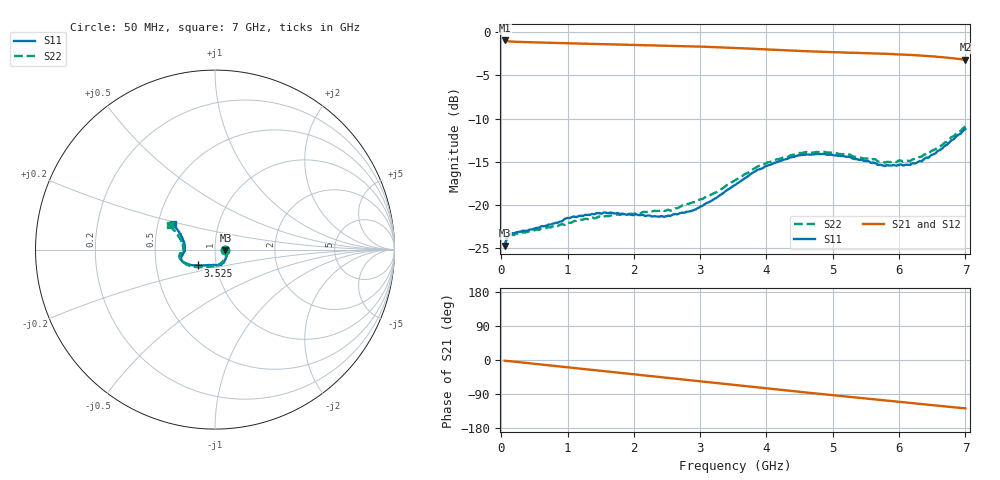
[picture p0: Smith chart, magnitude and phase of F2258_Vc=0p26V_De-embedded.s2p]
! Integrated Device Technology
! Corporate Headquarters
! 6024 Silver Creek Valley Road
! San Jose, CA 95138  USA
! Phone:  1-408-284-8200
! Toll Free:  1-800-223-1366
! Webpage:  http://www.idt.com/
! Timing and RF Division
! 515 Groton Road, Suite 102
! Westford, MA 01886-6024
! Device:  F2258
! Description: Voltage Variable RF Attenuator
! Frequency:  50.0 -  6000.00 MHz
! Package:  3x3 mm Thin QFN Plastic Package: 16 pin
! Ports:  2 RF, 2 DC
!  Pin  1  = NC
!  Pin  2  = NC
!  Pin  3  = RF2  = Port 2
!  Pin  4  = GND
!  Pin  5  = Vdd
!  Pin  6  = NC
!  Pin  7  = VCTRL
!  Pin  8  = NC
!  Pin  9  = GND
!  Pin 10  = RF1  = Port 1
!  Pin 11  = NC
!  Pin 12  = NC
!  Pin 13  = NC
!  Pin 14  = NC
!  Pin 15  = NC
!  Pin 16  = NC
! Vcntrl:  0.260 Volts
! Vdd:  +3.300 Volts
! Current:  1.080 mA
! Data:  The device was measured on a the F2258 evaluation board which has
!  individual transmission lines to the RF pins.  Data was collected
!  using a calibrated network analyzer.  The evaluation board was
!  de-embedded using a TRL calibration technique.
!  The reference plane is the edge of the package pin.
! Misc:  SN 10
!  Action Tracker AT0285
! Date Measured:  2014-12-10
! Date:  2016-01-13  MJV
! Note:
!  Integrated Device Technology supplies this data as a sample of measured
!  data at the package pin for this product.  Your particular data for this
!  product may vary.
!  Data was taken at 25 degrees C.
!  Integrated Device Technology reserves the right to change this data at anytime.
!Freq_(GHz)  S11M_(dB)  S11P_(deg)  S21M_(dB)  S21P_(deg)  S12M_(dB)  S12P_(deg)  S22M_(dB)  S22P_(deg)
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# GHz S dB R 50
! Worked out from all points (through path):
!   201 points, 50 MHz to 7 GHz, reference 50 ohm
!   highest |S21| = -0.97 dB at 50 MHz (marker M1); lowest = -3.2 dB at 7 GHz (marker M2)
!   group delay of S21, straight-line fit = 50.5 ps
!   lowest |S11| = -24.7 dB at 50 MHz (marker M3), VSWR 1.12, Z = 56.2 - j0.392 ohm
!   |S11| at or under -10 dB: start of sweep to end of sweep
!   |S22| runs from -24.8 to -10.9 dB; largest |S21 - S12| = 0.00035
!   S11 on the Smith chart (normalised r, x): 50 MHz: 1.12, -0.01; 3.525 GHz: 0.81, -0.15; 7 GHz: 0.60, +0.19
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0.05  -24.71 -3.4  -0.97 -1.9  -0.97 -1.9  -24.77 -3.0
0.08475  -23.74 -5.9  -1.04 -2.5  -1.04 -2.4  -23.83 -5.4
0.15425  -23.26 -9.1  -1.10 -3.6  -1.10 -3.6  -23.45 -9.4
0.71025  -22.27 -36.7  -1.23 -14.1  -1.23 -14.1  -22.56 -38.4
0.98825  -21.50 -50.5  -1.28 -19.3  -1.28 -19.3  -22.07 -54.4
1.2315  -21.27 -58.8  -1.34 -23.8  -1.34 -23.8  -21.70 -63.4
1.6485  -20.87 -70.4  -1.42 -31.4  -1.42 -31.4  -21.22 -76.4
2.37825  -21.36 -91.7  -1.55 -44.8  -1.55 -44.8  -20.69 -94.1
2.552  -21.27 -97.7  -1.58 -48.0  -1.58 -48.0  -20.66 -99.4
2.93425  -20.51 -114.3  -1.66 -55.1  -1.66 -55.1  -19.66 -112.7
3.525  -17.70 -137.2  -1.83 -66.2  -1.83 -66.2  -17.17 -135.4
4.0115  -15.44 -151.0  -2.01 -75.2  -2.01 -75.2  -15.09 -150.9
4.46325  -14.29 -159.4  -2.17 -83.4  -2.17 -83.4  -14.04 -162.0
4.7065  -14.16 -162.7  -2.24 -87.7  -2.24 -87.7  -13.94 -166.2
5.15825  -14.33 -168.2  -2.36 -95.6  -2.36 -95.6  -14.11 -173.1
5.64475  -15.17 -176.3  -2.48 -104.0  -2.48 -104.0  -14.74 -179.4
5.6795  -15.37 -176.4  -2.48 -104.6  -2.48 -104.6  -14.99 -179.6
5.85325  -15.43 179.4  -2.53 -107.8  -2.53 -107.8  -15.03 175.7
6.166  -15.37 171.6  -2.64 -113.4  -2.64 -113.4  -14.94 169.8
6.33975  -14.96 165.2  -2.72 -116.5  -2.72 -116.5  -14.40 165.4
6.722  -13.04 153.5  -2.95 -123.1  -2.96 -123.1  -12.69 156.4
7  -11.22 148.1  -3.20 -127.4  -3.20 -127.4  -10.90 151.5
